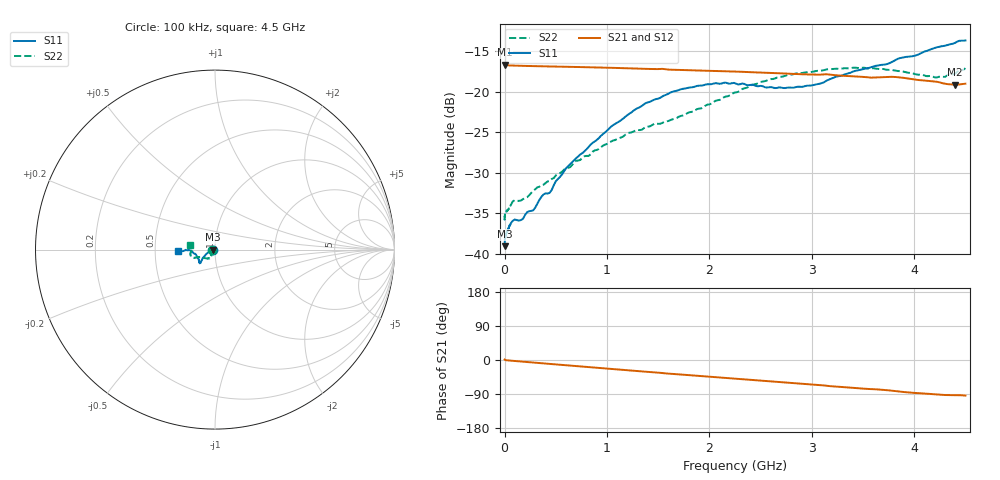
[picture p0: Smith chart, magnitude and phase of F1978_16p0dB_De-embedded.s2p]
! Integrated Device Technology
! Corporate Headquarters
! 6024 Silver Creek Valley Road
! San Jose, CA 95138  USA
! Phone:  1-408-284-8200
! Toll Free:  1-800-223-1366
! Webpage:  http://www.idt.com/
! Timing and RF Division
! 515 Groton Road, Suite 102
! Westford, MA 01886-6024
! Device:  F1978
! Description: 6-bit, 75 ohm, 0.5 dB Digital Step Attenuator
! Frequency:  5.0 MHz -  3.00 GHz
! Package:  4x4 mm QFN Plastic Package: 20 pin
! Ports:  2 RF, 11 DC
!  Pin  1  = D5 (16 dB)
!  Pin  2  = RF1  =  Port 1
!  Pin  3  = Serial Data In (DATA)
!  Pin  4  = Serial Clock (CLK)
!  Pin  5  = Serial Latch Enable (LE)
!  Pin  6  = VDD
!  Pin  7  = NC
!  Pin  8  = NC
!  Pin  9  = NC
!  Pin 10  = GND
!  Pin 11  = GND
!  Pin 12  = NC
!  Pin 13  = VMODE
!  Pin 14  = RF2  =  Port 2
!  Pin 15  = D4 (8 dB)
!  Pin 16  = D3 (4 dB)
!  Pin 17  = D2 (2 dB)
!  Pin 18  = NC
!  Pin 19  = D1 (1 dB)
!  Pin 20  = D0 (0.5 dB)
! State:  32
! Atten State:  16.0 dB
! Voltage:  +3.30 Volts
! Current:  0.593 mA
! Data:  The device was measured on a F1975 evaluation board which has
!  individual transmission lines to the RF pins.  Data was collected
!  using a calibrated network analyzer.  The evaluation board was
!  de-embedded using Automatic Fixture Removal (AFR).
!  The reference plane is the edge of the package pin.
! Misc:
!  Action Tracker AT0416
! Date Measured:  2018-02-08
! Date:  2018-03-26  MJV
! Note:
!  Integrated Device Technology supplies this data as a sample of measured
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# GHz S dB R 75
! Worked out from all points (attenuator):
!   291 points, 100 kHz to 4.5 GHz, reference 75 ohm
!   highest |S21| = -16.65 dB at 100 kHz (marker M1); lowest = -19.1 dB at 4.4 GHz (marker M2)
!   lowest |S11| = -39.1 dB at 100 kHz (marker M3), VSWR 1.02, Z = 73.3 - j0.00135 ohm
!   |S11| at or under -10 dB: start of sweep to end of sweep
!   |S22| runs from -35.8 to -17.0 dB; largest |S21 - S12| = 0.00017
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0.0001  -39.06 -180.0  -16.65 1.2  -16.64 1.2  -35.70 -178.8
0.002  -38.23 -177.2  -16.68 0.9  -16.68 0.8  -35.33 -177.0
0.012  -37.67 -176.3  -16.71 -0.5  -16.71 -0.5  -34.85 -175.0
0.08  -35.93 -170.4  -16.76 -2.1  -16.76 -2.1  -33.54 -165.0
0.16  -35.84 -167.9  -16.79 -4.0  -16.79 -4.0  -33.42 -152.2
0.28  -34.64 -167.6  -16.83 -6.7  -16.82 -6.7  -32.21 -142.1
0.36  -32.96 -167.5  -16.85 -8.5  -16.85 -8.5  -31.52 -134.0
0.44  -32.47 -165.2  -16.87 -10.3  -16.86 -10.3  -31.02 -128.2
0.6  -29.44 -162.7  -16.91 -13.8  -16.91 -13.8  -29.41 -123.7
0.76  -27.57 -156.6  -16.95 -17.4  -16.95 -17.4  -28.15 -121.3
1.06  -24.11 -150.0  -17.04 -24.0  -17.04 -24.0  -26.01 -119.5
1.38  -21.38 -144.7  -17.17 -31.0  -17.16 -31.0  -24.34 -125.4
1.52  -20.74 -141.8  -17.17 -33.9  -17.17 -33.8  -23.95 -128.9
1.88  -19.27 -138.1  -17.37 -41.6  -17.36 -41.6  -22.13 -143.7
2.26  -18.99 -139.5  -17.51 -49.6  -17.50 -49.6  -20.06 -154.8
2.58  -19.44 -148.9  -17.66 -56.3  -17.65 -56.3  -18.50 -157.7
3.02  -19.15 -165.8  -17.87 -65.2  -17.86 -65.2  -17.50 -160.8
3.42  -17.43 -176.6  -18.09 -73.9  -18.09 -73.9  -17.01 -166.9
3.76  -16.46 -178.4  -18.15 -80.3  -18.15 -80.3  -17.30 -173.5
4.2  -14.58 -177.2  -18.73 -90.6  -18.73 -90.6  -18.21 175.1
4.4  -13.95 -176.1  -19.13 -92.8  -19.12 -92.8  -17.76 172.0
4.5  -13.66 -178.0  -19.00 -93.9  -18.99 -93.9  -17.08 170.5
